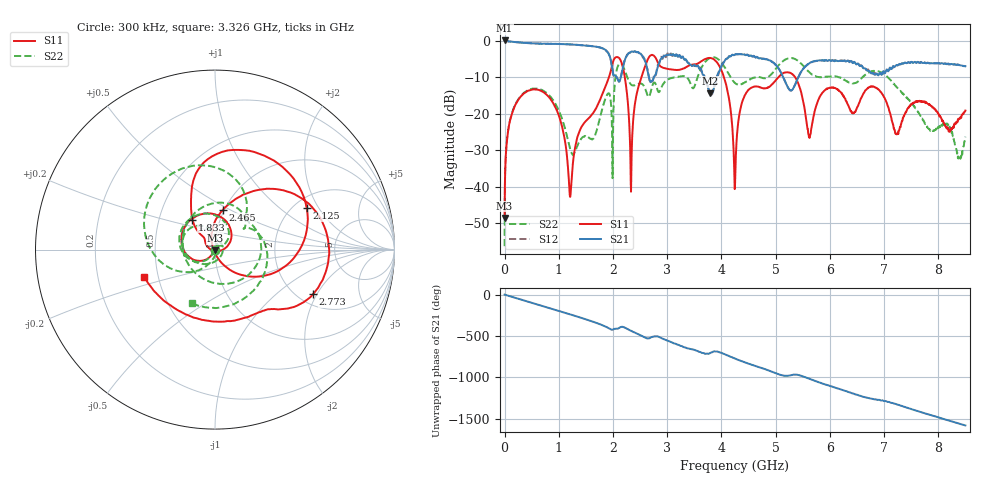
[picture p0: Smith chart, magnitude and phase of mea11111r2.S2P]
!Agilent Technologies,E5071B,MY42402595,A.08.01
!Date: Tue Jan 02 10:21:52 2001
!Data & Calibration Information:
!Freq	S11:SOLT2(ON)	S21:SOLT2(ON)	S12:SOLT2(ON)	S22:SOLT2(ON)
# Hz S dB R 50
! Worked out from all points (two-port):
!   1601 points, 300 kHz to 8.5 GHz, reference 50 ohm
!   highest |S21| = 0.02 dB at 300 kHz (marker M1); lowest = -14.4 dB at 3.788 GHz (marker M2)
!   |S21| within 3 dB of the highest: start of sweep to 1.89 GHz; 2.391 GHz to 2.409 GHz (18.64 MHz wide, 0.777 % of centre)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
!   lowest |S11| = -48.6 dB at 300 kHz (marker M3), VSWR 1.01, Z = 50 - j0.371 ohm
!   |S11| at or under -10 dB: start of sweep to 1.926 GHz; 4.047 GHz to 5.054 GHz (1.007 GHz wide, 22.1 % of centre); 5.355 GHz to end of sweep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
!   |S22| runs from -56.3 to -4.5 dB; largest |S21 - S12| = 0.044
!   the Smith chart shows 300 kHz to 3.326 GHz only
!   S11 on the Smith chart (normalised r, x): 300 kHz: 1.00, -0.01; 1.833 GHz: 0.74, +0.26; 2.125 GHz: 2.35, +1.58; 2.465 GHz: 0.98, +0.46; 2.773 GHz: 2.39, -1.86; 3.326 GHz: 0.42, -0.15
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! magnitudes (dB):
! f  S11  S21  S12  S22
! 300 kHz  -48.6  0.0  0.0  -56.3
! 85.3 MHz  -22.9  -0.2  -0.2  -22.8
! 350.9 MHz  -14.5  -0.6  -0.6  -14.4
! 924.6 MHz  -17.9  -0.9  -0.9  -17.0
! 1.212 GHz  -42.8  -1.0  -1.1  -29.8
! 1.419 GHz  -23.6  -1.3  -1.3  -26.8
! 1.833 GHz  -13.6  -2.3  -2.4  -17.1
! 2.125 GHz  -5.0  -11.0  -11.0  -6.3
! 2.332 GHz  -41.4  -3.1  -3.1  -12.1
! 2.465 GHz  -12.9  -3.2  -3.2  -11.8
! 2.773 GHz  -4.4  -9.5  -9.4  -11.6
! 2.837 GHz  -6.3  -6.6  -6.6  -14.1
! 3.326 GHz  -7.5  -5.2  -5.1  -9.8
! 3.788 GHz  -4.8  -14.4  -14.0  -4.8
! 4.08 GHz  -11.7  -5.1  -5.2  -7.8
! 4.25 GHz  -39.9  -3.8  -3.8  -11.7
! 4.452 GHz  -14.4  -4.0  -4.0  -11.3
! 5.159 GHz  -8.8  -10.7  -10.6  -5.4
! 5.669 GHz  -23.2  -5.9  -5.9  -9.3
! 6.009 GHz  -12.9  -5.5  -5.5  -9.9
! 7.087 GHz  -18.6  -8.2  -8.1  -10.4
! 8.5 GHz  -19.2  -7.0  -7.0  -26.3
